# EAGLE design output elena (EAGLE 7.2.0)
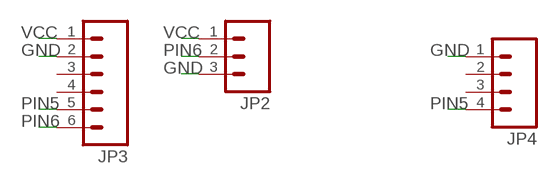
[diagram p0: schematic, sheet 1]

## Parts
JP2  M031X03_NO_SILK  [1X03_NO_SILK]
JP3  M06LONGPADS  [1X06_LONGPADS]
JP4  M04LONGPADS  [1X04_LONGPADS]

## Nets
GND: JP2.3 JP3.2 JP4.1
PIN5: JP3.5 JP4.4
PIN6: JP2.2 JP3.6
VCC: JP2.1 JP3.1
Unconnected: JP3.3 JP3.4 JP4.2 JP4.3

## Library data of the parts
JP2 = 01_SparkFun:M03: Header 3 Standard 3-pin 0.1" header. Use with straight break away headers (SKU : PRT-00116), right angle break away headers (PRT-00553), swiss pins (PRT-00743), machine pins (PRT-00117), and female headers (PRT-00115). Molex polarized connector foot print use with SKU : PRT-08232 with associated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
JP3 = 01_SparkFun:M06: Header 6 Standard 6-pin 0.1" header. Use with straight break away headers (SKU : PRT-00116), right angle break away headers (PRT-00553), swiss pins (PRT-00743), machine pins (PRT-00117), and female headers (PRT-00115). Molex polarized connector foot print use with SKU : PRT-08094 with associated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
JP4 = 01_SparkFun:M04: Header 4 Standard 4-pin 0.1" header. Use with straight break away headers (SKU : PRT-00116), right angle break away headers (PRT-00553), swiss pins (PRT-00743), machine pins (PRT-00117), and female headers (PRT-00115). Molex polarized connector foot print use with SKU : PRT-08231 with associated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

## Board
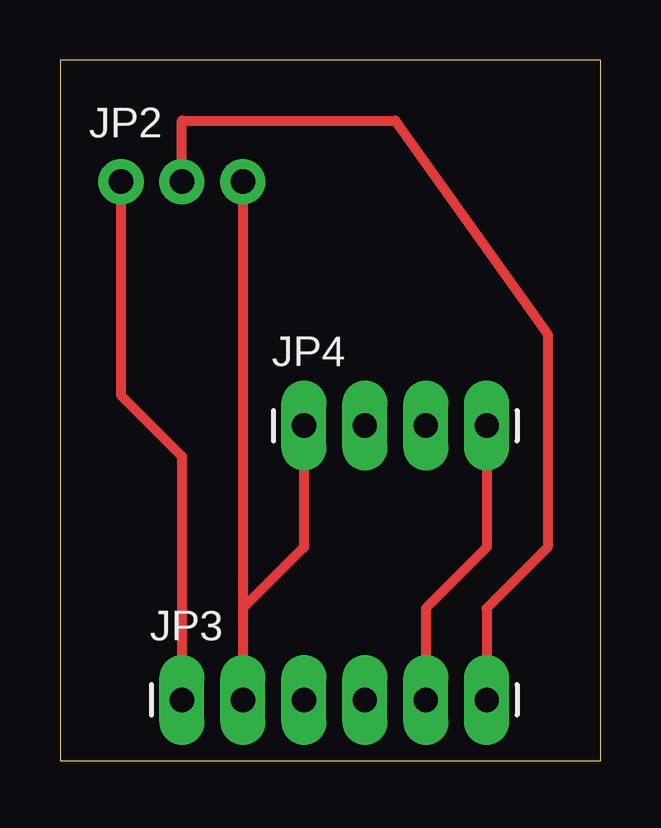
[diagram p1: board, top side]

Size 22.53 x 29.2 mm. Coordinates in mm from the lower left corner, seen from the top.
Outline: 0,0 22.53,0 22.53,29.2 0,29.2 0,0
Copper layers (1*16): Top 0.035mm / dielectric 1.5mm / Bottom 0.035mm
Design rules "default": minimum track width 10mil, minimum drill 24mil, track to track 8mil, track to pad 8mil, pad to pad 8mil, via to via 8mil, smd to smd 8mil, copper to edge 40mil, drill to drill 8mil, minimum pad ring 10mil, minimum via ring 8mil, stop-mask expansion 4mil, vias tented up to drill 0mil, thermal gap 10mil

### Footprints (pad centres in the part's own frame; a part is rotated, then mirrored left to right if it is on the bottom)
1X03_NO_SILK = drill 1.016 pad 1.88: 1 0,0; 2 2.54,0; 3 5.08,0
1X06_LONGPADS = drill 1.016 pad 1.88 long: 1 0,0; 2 2.54,0; 3 5.08,0; 4 7.62,0; 5 10.16,0; 6 12.7,0
1X04_LONGPADS = drill 1.016 pad 1.88 long: 1 0,0; 2 2.54,0; 3 5.08,0; 4 7.62,0

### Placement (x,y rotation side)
JP2  2.54,24.13 0 top
JP3  5.08,2.54 0 top
JP4  10.16,13.97 0 top

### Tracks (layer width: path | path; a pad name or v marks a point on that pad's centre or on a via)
GND
  Top 0.406: JP2.3 7.62,6.35 | 7.62,6.35 JP3.2 | JP4.1 10.16,8.89 7.62,6.35
PIN5
  Top 0.406: JP4.4 17.78,8.89 15.24,6.35 JP3.5
PIN6
  Top 0.406: JP2.2 5.08,26.67 13.97,26.67 20.32,17.78 20.32,8.89 17.78,6.35 JP3.6
VCC
  Top 0.406: JP2.1 2.54,15.24 5.08,12.7 JP3.1

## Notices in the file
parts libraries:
01_SparkFun: Licensing: CC v3.0 Share-Alike You are welcome to use this library for commercial purposes.
